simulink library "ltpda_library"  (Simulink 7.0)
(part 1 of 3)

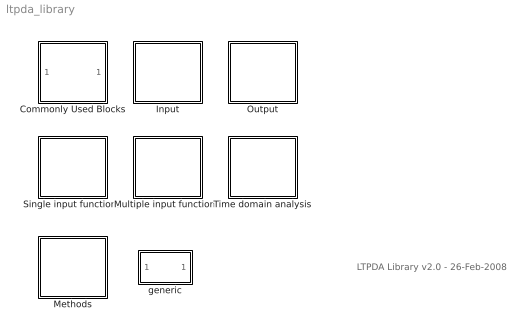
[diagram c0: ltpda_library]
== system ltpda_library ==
  note: LTPDA Library v2.0 - 26-Feb-2008
  Commonly Used Blocks : Subsystem
  Input : Subsystem
  Methods : Subsystem  Tag=subsystem  AncestorBlock=libraryBase/SubSystName
  Multiple input functions : Subsystem
  Output : Subsystem
  Single input functions : Subsystem
  Time domain analysis : Subsystem
  generic : Subsystem  Tag=function

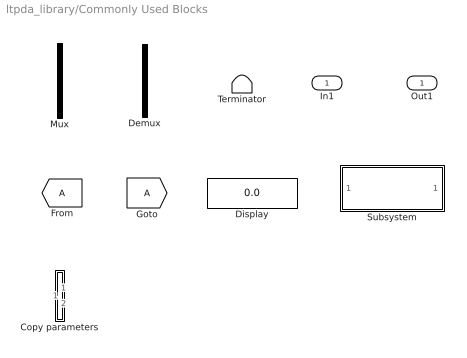
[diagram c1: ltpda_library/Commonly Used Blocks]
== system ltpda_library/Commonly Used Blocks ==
  In1 : Inport  OutDataType=sfix(16)  OutScaling=2^0
  Copy parameters : Subsystem
  Demux : Demux  Tag=demux  Outputs=2
  Display : Display
  Mux : Mux  Tag=mux  Inputs=2
  Subsystem : Subsystem
  Terminator : Terminator
  Out1 : Outport  OutDataType=sfix(16)  OutScaling=2^0

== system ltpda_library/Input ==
  AO from plist : Subsystem  Tag=freepl
  Object from list : Subsystem  Tag=input

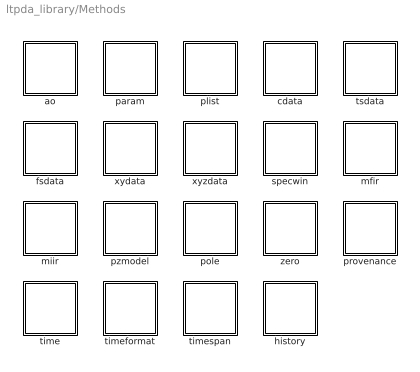
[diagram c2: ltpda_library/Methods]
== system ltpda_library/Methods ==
  ao : Subsystem  Tag=subsystem  AncestorBlock=libraryBase/SubSystName
  cdata : Subsystem  Tag=subsystem  AncestorBlock=libraryBase/SubSystName
  fsdata : Subsystem  Tag=subsystem  AncestorBlock=libraryBase/SubSystName
  history : Subsystem  Tag=subsystem  AncestorBlock=libraryBase/SubSystName
  mfir : Subsystem  Tag=subsystem  AncestorBlock=libraryBase/SubSystName
  miir : Subsystem  Tag=subsystem  AncestorBlock=libraryBase/SubSystName
  param : Subsystem  Tag=subsystem  AncestorBlock=libraryBase/SubSystName
  plist : Subsystem  Tag=subsystem  AncestorBlock=libraryBase/SubSystName
  pole : Subsystem  Tag=subsystem  AncestorBlock=libraryBase/SubSystName
  provenance : Subsystem  Tag=subsystem  AncestorBlock=libraryBase/SubSystName
  pzmodel : Subsystem  Tag=subsystem  AncestorBlock=libraryBase/SubSystName
  specwin : Subsystem  Tag=subsystem  AncestorBlock=libraryBase/SubSystName
  time : Subsystem  Tag=subsystem  AncestorBlock=libraryBase/SubSystName
  timeformat : Subsystem  Tag=subsystem  AncestorBlock=libraryBase/SubSystName
  timespan : Subsystem  Tag=subsystem  AncestorBlock=libraryBase/SubSystName
  tsdata : Subsystem  Tag=subsystem  AncestorBlock=libraryBase/SubSystName
  xydata : Subsystem  Tag=subsystem  AncestorBlock=libraryBase/SubSystName
  xyzdata : Subsystem  Tag=subsystem  AncestorBlock=libraryBase/SubSystName
  zero : Subsystem  Tag=subsystem  AncestorBlock=libraryBase/SubSystName

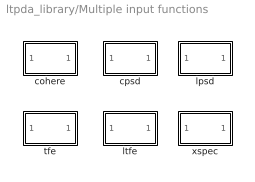
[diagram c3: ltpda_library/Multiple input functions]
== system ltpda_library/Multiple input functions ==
  cohere : Subsystem  Tag=function
  cpsd : Subsystem  Tag=function
  lpsd : Subsystem  Tag=function
  ltfe : Subsystem  Tag=function
  tfe : Subsystem  Tag=function
  xspec : Subsystem  Tag=function

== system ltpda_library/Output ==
  Plot : Subsystem
  Save Result : Subsystem
  iPlot : Subsystem

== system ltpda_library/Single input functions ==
  compute_f : Subsystem  Tag=function
  linedetect : Subsystem  Tag=function
  nfest : Subsystem  Tag=function
  psd : Subsystem  Tag=function
  pwelch : Subsystem  Tag=function
  rms : Subsystem  Tag=function

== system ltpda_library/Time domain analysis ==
  chkts : Subsystem  Tag=function
  polydetrend : Subsystem  Tag=function
  timedomainfit : Subsystem  Tag=function

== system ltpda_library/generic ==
  In1 : Inport  OutDataType=sfix(16)  OutScaling=2^0
  generic : M-S-Function  Tag=generic  FunctionName=ltpdasim
  Out1 : Outport  OutDataType=sfix(16)  OutScaling=2^0
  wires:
  generic/1 -> Out1/1
  In1/1 -> generic/1

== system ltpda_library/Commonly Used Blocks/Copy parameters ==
  In1 : Inport  OutDataType=sfix(16)  OutScaling=2^0
  In2 : Inport  Port=2  OutDataType=sfix(16)  OutScaling=2^0
  copyparam : M-S-Function  FunctionName=g_copyparams
  Out1 : Outport  OutDataType=sfix(16)  OutScaling=2^0
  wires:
  copyparam/1 -> Out1/1
  In1/1 -> copyparam/1
  In2/1 -> copyparam/2

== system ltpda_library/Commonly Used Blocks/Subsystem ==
  In1 : Inport  OutDataType=sfix(16)  OutScaling=2^0
  Out1 : Outport  OutDataType=sfix(16)  OutScaling=2^0
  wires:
  In1/1 -> Out1/1

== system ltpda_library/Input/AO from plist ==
  pl2ao : M-S-Function  FunctionName=g_pl2ao
  Out1 : Outport  OutDataType=sfix(16)  OutScaling=2^0
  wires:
  pl2ao/1 -> Out1/1

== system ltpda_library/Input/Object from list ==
  Input : Constant  Value=0  OutDataType=sfix(16)  OutScaling=2^0
  Input AO : Outport  OutDataType=sfix(16)  OutScaling=2^0
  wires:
  Input/1 -> Input AO/1

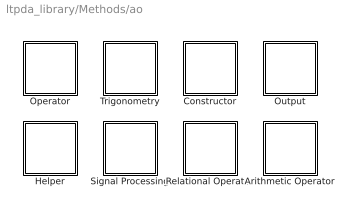
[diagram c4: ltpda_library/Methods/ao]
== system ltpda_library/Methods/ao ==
  Arithmetic Operator : Subsystem  Tag=subsystem  AncestorBlock=libraryBase/SubSystName
  Constructor : Subsystem  Tag=subsystem  AncestorBlock=libraryBase/SubSystName
  Helper : Subsystem  Tag=subsystem  AncestorBlock=libraryBase/SubSystName
  Operator : Subsystem  Tag=subsystem  AncestorBlock=libraryBase/SubSystName
  Output : Subsystem  Tag=subsystem  AncestorBlock=libraryBase/SubSystName
  Relational Operator : Subsystem  Tag=subsystem  AncestorBlock=libraryBase/SubSystName
  Signal Processing : Subsystem  Tag=subsystem  AncestorBlock=libraryBase/SubSystName
  Trigonometry : Subsystem  Tag=subsystem  AncestorBlock=libraryBase/SubSystName

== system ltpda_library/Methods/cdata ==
  Constructor : Subsystem  Tag=subsystem  AncestorBlock=libraryBase/SubSystName
  Helper : Subsystem  Tag=subsystem  AncestorBlock=libraryBase/SubSystName
  Output : Subsystem  Tag=subsystem  AncestorBlock=libraryBase/SubSystName
  Relational Operator : Subsystem  Tag=subsystem  AncestorBlock=libraryBase/SubSystName

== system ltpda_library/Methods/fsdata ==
  Constructor : Subsystem  Tag=subsystem  AncestorBlock=libraryBase/SubSystName
  Helper : Subsystem  Tag=subsystem  AncestorBlock=libraryBase/SubSystName
  Output : Subsystem  Tag=subsystem  AncestorBlock=libraryBase/SubSystName
  Relational Operator : Subsystem  Tag=subsystem  AncestorBlock=libraryBase/SubSystName

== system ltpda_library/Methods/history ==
  Constructor : Subsystem  Tag=subsystem  AncestorBlock=libraryBase/SubSystName
  Helper : Subsystem  Tag=subsystem  AncestorBlock=libraryBase/SubSystName
  Output : Subsystem  Tag=subsystem  AncestorBlock=libraryBase/SubSystName
  Relational Operator : Subsystem  Tag=subsystem  AncestorBlock=libraryBase/SubSystName

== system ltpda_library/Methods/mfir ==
  Constructor : Subsystem  Tag=subsystem  AncestorBlock=libraryBase/SubSystName
  Helper : Subsystem  Tag=subsystem  AncestorBlock=libraryBase/SubSystName
  Output : Subsystem  Tag=subsystem  AncestorBlock=libraryBase/SubSystName
  Relational Operator : Subsystem  Tag=subsystem  AncestorBlock=libraryBase/SubSystName
  Signal Processing : Subsystem  Tag=subsystem  AncestorBlock=libraryBase/SubSystName

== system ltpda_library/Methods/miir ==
  Constructor : Subsystem  Tag=subsystem  AncestorBlock=libraryBase/SubSystName
  Helper : Subsystem  Tag=subsystem  AncestorBlock=libraryBase/SubSystName
  Output : Subsystem  Tag=subsystem  AncestorBlock=libraryBase/SubSystName
  Relational Operator : Subsystem  Tag=subsystem  AncestorBlock=libraryBase/SubSystName
  Signal Processing : Subsystem  Tag=subsystem  AncestorBlock=libraryBase/SubSystName

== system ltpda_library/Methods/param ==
  Constructor : Subsystem  Tag=subsystem  AncestorBlock=libraryBase/SubSystName
  Helper : Subsystem  Tag=subsystem  AncestorBlock=libraryBase/SubSystName
  Operator : Subsystem  Tag=subsystem  AncestorBlock=libraryBase/SubSystName
  Output : Subsystem  Tag=subsystem  AncestorBlock=libraryBase/SubSystName
  Relational Operator : Subsystem  Tag=subsystem  AncestorBlock=libraryBase/SubSystName

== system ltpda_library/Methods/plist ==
  Constructor : Subsystem  Tag=subsystem  AncestorBlock=libraryBase/SubSystName
  Helper : Subsystem  Tag=subsystem  AncestorBlock=libraryBase/SubSystName
  Output : Subsystem  Tag=subsystem  AncestorBlock=libraryBase/SubSystName
  Relational Operator : Subsystem  Tag=subsystem  AncestorBlock=libraryBase/SubSystName
  Signal Processing : Subsystem  Tag=subsystem  AncestorBlock=libraryBase/SubSystName

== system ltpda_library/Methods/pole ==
  Constructor : Subsystem  Tag=subsystem  AncestorBlock=libraryBase/SubSystName
  Helper : Subsystem  Tag=subsystem  AncestorBlock=libraryBase/SubSystName
  Output : Subsystem  Tag=subsystem  AncestorBlock=libraryBase/SubSystName
  Relational Operator : Subsystem  Tag=subsystem  AncestorBlock=libraryBase/SubSystName
  Signal Processing : Subsystem  Tag=subsystem  AncestorBlock=libraryBase/SubSystName

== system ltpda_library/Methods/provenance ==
  Constructor : Subsystem  Tag=subsystem  AncestorBlock=libraryBase/SubSystName
  Helper : Subsystem  Tag=subsystem  AncestorBlock=libraryBase/SubSystName
  Output : Subsystem  Tag=subsystem  AncestorBlock=libraryBase/SubSystName
  Relational Operator : Subsystem  Tag=subsystem  AncestorBlock=libraryBase/SubSystName

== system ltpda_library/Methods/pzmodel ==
  Constructor : Subsystem  Tag=subsystem  AncestorBlock=libraryBase/SubSystName
  Helper : Subsystem  Tag=subsystem  AncestorBlock=libraryBase/SubSystName
  Operator : Subsystem  Tag=subsystem  AncestorBlock=libraryBase/SubSystName
  Output : Subsystem  Tag=subsystem  AncestorBlock=libraryBase/SubSystName
  Relational Operator : Subsystem  Tag=subsystem  AncestorBlock=libraryBase/SubSystName
  Signal Processing : Subsystem  Tag=subsystem  AncestorBlock=libraryBase/SubSystName

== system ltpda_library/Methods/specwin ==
  Constructor : Subsystem  Tag=subsystem  AncestorBlock=libraryBase/SubSystName
  Helper : Subsystem  Tag=subsystem  AncestorBlock=libraryBase/SubSystName
  Output : Subsystem  Tag=subsystem  AncestorBlock=libraryBase/SubSystName
  Relational Operator : Subsystem  Tag=subsystem  AncestorBlock=libraryBase/SubSystName

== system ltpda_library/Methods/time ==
  Arithmetic Operator : Subsystem  Tag=subsystem  AncestorBlock=libraryBase/SubSystName
  Constructor : Subsystem  Tag=subsystem  AncestorBlock=libraryBase/SubSystName
  Helper : Subsystem  Tag=subsystem  AncestorBlock=libraryBase/SubSystName
  Output : Subsystem  Tag=subsystem  AncestorBlock=libraryBase/SubSystName
  Relational Operator : Subsystem  Tag=subsystem  AncestorBlock=libraryBase/SubSystName

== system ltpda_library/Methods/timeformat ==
  Constructor : Subsystem  Tag=subsystem  AncestorBlock=libraryBase/SubSystName
  Helper : Subsystem  Tag=subsystem  AncestorBlock=libraryBase/SubSystName
  Output : Subsystem  Tag=subsystem  AncestorBlock=libraryBase/SubSystName
  Relational Operator : Subsystem  Tag=subsystem  AncestorBlock=libraryBase/SubSystName

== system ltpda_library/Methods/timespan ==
  Constructor : Subsystem  Tag=subsystem  AncestorBlock=libraryBase/SubSystName
  Helper : Subsystem  Tag=subsystem  AncestorBlock=libraryBase/SubSystName
  Output : Subsystem  Tag=subsystem  AncestorBlock=libraryBase/SubSystName
  Relational Operator : Subsystem  Tag=subsystem  AncestorBlock=libraryBase/SubSystName

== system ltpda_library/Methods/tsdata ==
  Constructor : Subsystem  Tag=subsystem  AncestorBlock=libraryBase/SubSystName
  Helper : Subsystem  Tag=subsystem  AncestorBlock=libraryBase/SubSystName
  Output : Subsystem  Tag=subsystem  AncestorBlock=libraryBase/SubSystName
  Relational Operator : Subsystem  Tag=subsystem  AncestorBlock=libraryBase/SubSystName

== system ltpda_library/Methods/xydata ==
  Constructor : Subsystem  Tag=subsystem  AncestorBlock=libraryBase/SubSystName
  Helper : Subsystem  Tag=subsystem  AncestorBlock=libraryBase/SubSystName
  Output : Subsystem  Tag=subsystem  AncestorBlock=libraryBase/SubSystName
  Relational Operator : Subsystem  Tag=subsystem  AncestorBlock=libraryBase/SubSystName

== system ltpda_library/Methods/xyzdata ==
  Constructor : Subsystem  Tag=subsystem  AncestorBlock=libraryBase/SubSystName
  Helper : Subsystem  Tag=subsystem  AncestorBlock=libraryBase/SubSystName
  Output : Subsystem  Tag=subsystem  AncestorBlock=libraryBase/SubSystName
  Relational Operator : Subsystem  Tag=subsystem  AncestorBlock=libraryBase/SubSystName

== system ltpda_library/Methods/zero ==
  Constructor : Subsystem  Tag=subsystem  AncestorBlock=libraryBase/SubSystName
  Helper : Subsystem  Tag=subsystem  AncestorBlock=libraryBase/SubSystName
  Output : Subsystem  Tag=subsystem  AncestorBlock=libraryBase/SubSystName
  Relational Operator : Subsystem  Tag=subsystem  AncestorBlock=libraryBase/SubSystName
  Signal Processing : Subsystem  Tag=subsystem  AncestorBlock=libraryBase/SubSystName

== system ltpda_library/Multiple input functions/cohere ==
  In1 : Inport  OutDataType=sfix(16)  OutScaling=2^0
  ltpda_cohere : M-S-Function  Tag=ltpda_cohere  FunctionName=ltpdasim
  Out1 : Outport  OutDataType=sfix(16)  OutScaling=2^0
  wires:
  ltpda_cohere/1 -> Out1/1
  In1/1 -> ltpda_cohere/1

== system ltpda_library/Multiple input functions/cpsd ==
  In1 : Inport  OutDataType=sfix(16)  OutScaling=2^0
  ltpda_cpsd : M-S-Function  Tag=ltpda_cpsd  FunctionName=ltpdasim
  Out1 : Outport  OutDataType=sfix(16)  OutScaling=2^0
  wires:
  ltpda_cpsd/1 -> Out1/1
  In1/1 -> ltpda_cpsd/1

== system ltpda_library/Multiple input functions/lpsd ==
  In1 : Inport  OutDataType=sfix(16)  OutScaling=2^0
  ltpda_lpsd : M-S-Function  Tag=ltpda_lpsd  FunctionName=ltpdasim
  Out1 : Outport  OutDataType=sfix(16)  OutScaling=2^0
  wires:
  In1/1 -> ltpda_lpsd/1
  ltpda_lpsd/1 -> Out1/1

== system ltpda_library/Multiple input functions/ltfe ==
  In1 : Inport  OutDataType=sfix(16)  OutScaling=2^0
  ltpda_ltfe : M-S-Function  Tag=ltpda_ltfe  FunctionName=ltpdasim
  Out1 : Outport  OutDataType=sfix(16)  OutScaling=2^0
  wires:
  In1/1 -> ltpda_ltfe/1
  ltpda_ltfe/1 -> Out1/1

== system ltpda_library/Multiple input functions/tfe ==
  In1 : Inport  OutDataType=sfix(16)  OutScaling=2^0
  ltpda_tfe : M-S-Function  Tag=ltpda_tfe  FunctionName=ltpdasim
  Out1 : Outport  OutDataType=sfix(16)  OutScaling=2^0
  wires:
  ltpda_tfe/1 -> Out1/1
  In1/1 -> ltpda_tfe/1

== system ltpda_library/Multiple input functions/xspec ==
  In1 : Inport  OutDataType=sfix(16)  OutScaling=2^0
  ltpda_xspec : M-S-Function  Tag=ltpda_xspec  FunctionName=ltpdasim
  Out1 : Outport  OutDataType=sfix(16)  OutScaling=2^0
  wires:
  ltpda_xspec/1 -> Out1/1
  In1/1 -> ltpda_xspec/1

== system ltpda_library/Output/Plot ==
  In1 : Inport  OutDataType=sfix(16)  OutScaling=2^0
  plot : M-S-Function  FunctionName=g_plot
  Out1 : Outport  OutDataType=sfix(16)  OutScaling=2^0
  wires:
  plot/1 -> Out1/1
  In1/1 -> plot/1

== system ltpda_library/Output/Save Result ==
  In1 : Inport  OutDataType=sfix(16)  OutScaling=2^0
  save result : M-S-Function  FunctionName=g_saveresult
  Out1 : Outport  OutDataType=sfix(16)  OutScaling=2^0
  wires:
  In1/1 -> save result/1
  save result/1 -> Out1/1

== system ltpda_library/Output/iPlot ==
  In1 : Inport  OutDataType=sfix(16)  OutScaling=2^0
  iplot : M-S-Function  FunctionName=g_iplot
  Out1 : Outport  OutDataType=sfix(16)  OutScaling=2^0
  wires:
  In1/1 -> iplot/1
  iplot/1 -> Out1/1

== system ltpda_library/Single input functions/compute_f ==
  In1 : Inport  OutDataType=sfix(16)  OutScaling=2^0
  ltpda_compute_f : M-S-Function  Tag=ltpda_compute_f  FunctionName=ltpdasim
  Out1 : Outport  OutDataType=sfix(16)  OutScaling=2^0
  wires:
  ltpda_compute_f/1 -> Out1/1
  In1/1 -> ltpda_compute_f/1

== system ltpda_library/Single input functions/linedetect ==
  In1 : Inport  OutDataType=sfix(16)  OutScaling=2^0
  ltpda_linedetect : M-S-Function  Tag=ltpda_linedetect  FunctionName=ltpdasim
  Out1 : Outport  OutDataType=sfix(16)  OutScaling=2^0
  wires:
  In1/1 -> ltpda_linedetect/1
  ltpda_linedetect/1 -> Out1/1

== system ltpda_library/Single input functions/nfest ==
  In1 : Inport  OutDataType=sfix(16)  OutScaling=2^0
  ltpda_nfest : M-S-Function  Tag=ltpda_nfest  FunctionName=ltpdasim
  Out1 : Outport  OutDataType=sfix(16)  OutScaling=2^0
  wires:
  ltpda_nfest/1 -> Out1/1
  In1/1 -> ltpda_nfest/1

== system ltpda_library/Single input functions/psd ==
  In1 : Inport  OutDataType=sfix(16)  OutScaling=2^0
  ltpda_psd : M-S-Function  Tag=ltpda_psd  FunctionName=ltpdasim
  Out1 : Outport  OutDataType=sfix(16)  OutScaling=2^0
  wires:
  ltpda_psd/1 -> Out1/1
  In1/1 -> ltpda_psd/1

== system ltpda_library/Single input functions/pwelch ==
  In1 : Inport  OutDataType=sfix(16)  OutScaling=2^0
  ltpda_pwelch : M-S-Function  Tag=ltpda_pwelch  FunctionName=ltpdasim
  Out1 : Outport  OutDataType=sfix(16)  OutScaling=2^0
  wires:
  In1/1 -> ltpda_pwelch/1
  ltpda_pwelch/1 -> Out1/1

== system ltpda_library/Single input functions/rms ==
  In1 : Inport  OutDataType=sfix(16)  OutScaling=2^0
  ltpda_rms : M-S-Function  Tag=ltpda_rms  FunctionName=ltpdasim
  Out1 : Outport  OutDataType=sfix(16)  OutScaling=2^0
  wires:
  In1/1 -> ltpda_rms/1
  ltpda_rms/1 -> Out1/1

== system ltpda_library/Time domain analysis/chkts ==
  In1 : Inport  OutDataType=sfix(16)  OutScaling=2^0
  ltpda_chkts : M-S-Function  Tag=ltpda_chkts  FunctionName=ltpdasim
  Out1 : Outport  OutDataType=sfix(16)  OutScaling=2^0
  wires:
  ltpda_chkts/1 -> Out1/1
  In1/1 -> ltpda_chkts/1

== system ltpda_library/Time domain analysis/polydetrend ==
  In1 : Inport  OutDataType=sfix(16)  OutScaling=2^0
  ltpda_polydetrend : M-S-Function  Tag=ltpda_polydetrend  FunctionName=ltpdasim
  Out1 : Outport  OutDataType=sfix(16)  OutScaling=2^0
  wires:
  In1/1 -> ltpda_polydetrend/1
  ltpda_polydetrend/1 -> Out1/1

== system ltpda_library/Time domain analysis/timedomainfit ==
  In1 : Inport  OutDataType=sfix(16)  OutScaling=2^0
  ltpda_timedomainfit : M-S-Function  Tag=ltpda_timedomainfit  FunctionName=ltpdasim
  Out1 : Outport  OutDataType=sfix(16)  OutScaling=2^0
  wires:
  ltpda_timedomainfit/1 -> Out1/1
  In1/1 -> ltpda_timedomainfit/1

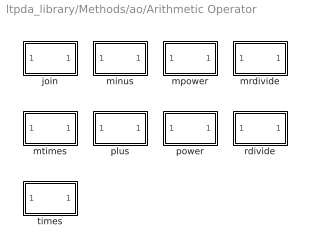
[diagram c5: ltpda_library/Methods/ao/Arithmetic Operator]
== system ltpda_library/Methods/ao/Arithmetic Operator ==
  join : Subsystem  Tag=method ao  AncestorBlock=libraryBase/function
  minus : Subsystem  Tag=method ao  AncestorBlock=libraryBase/function
  mpower : Subsystem  Tag=method ao  AncestorBlock=libraryBase/function
  mrdivide : Subsystem  Tag=method ao  AncestorBlock=libraryBase/function
  mtimes : Subsystem  Tag=method ao  AncestorBlock=libraryBase/function
  plus : Subsystem  Tag=method ao  AncestorBlock=libraryBase/function
  power : Subsystem  Tag=method ao  AncestorBlock=libraryBase/function
  rdivide : Subsystem  Tag=method ao  AncestorBlock=libraryBase/function
  times : Subsystem  Tag=method ao  AncestorBlock=libraryBase/function

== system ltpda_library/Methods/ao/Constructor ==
  ao : Subsystem  Tag=method ao  AncestorBlock=libraryBase/constructor

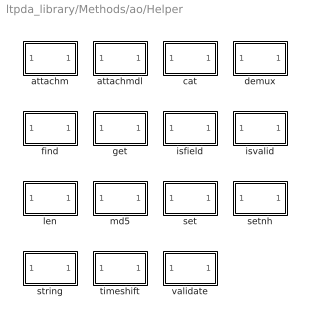
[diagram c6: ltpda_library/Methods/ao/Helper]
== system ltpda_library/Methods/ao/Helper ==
  attachm : Subsystem  Tag=method ao  AncestorBlock=libraryBase/function
  attachmdl : Subsystem  Tag=method ao  AncestorBlock=libraryBase/function
  cat : Subsystem  Tag=method ao  AncestorBlock=libraryBase/function
  demux : Subsystem  Tag=method ao  AncestorBlock=libraryBase/function
  find : Subsystem  Tag=method ao  AncestorBlock=libraryBase/function
  get : Subsystem  Tag=method ao  AncestorBlock=libraryBase/function
  isfield : Subsystem  Tag=method ao  AncestorBlock=libraryBase/function
  isvalid : Subsystem  Tag=method ao  AncestorBlock=libraryBase/function
  len : Subsystem  Tag=method ao  AncestorBlock=libraryBase/function
  md5 : Subsystem  Tag=method ao  AncestorBlock=libraryBase/function
  set : Subsystem  Tag=method ao  AncestorBlock=libraryBase/function
  setnh : Subsystem  Tag=method ao  AncestorBlock=libraryBase/function
  string : Subsystem  Tag=method ao  AncestorBlock=libraryBase/function
  timeshift : Subsystem  Tag=method ao  AncestorBlock=libraryBase/function
  validate : Subsystem  Tag=method ao  AncestorBlock=libraryBase/function

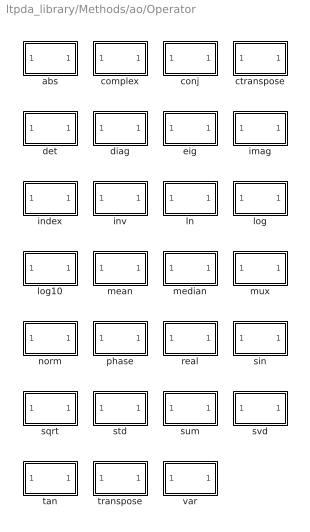
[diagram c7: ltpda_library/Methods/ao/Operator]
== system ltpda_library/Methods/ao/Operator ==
  abs : Subsystem  Tag=method ao  AncestorBlock=libraryBase/function
  complex : Subsystem  Tag=method ao  AncestorBlock=libraryBase/function
  conj : Subsystem  Tag=method ao  AncestorBlock=libraryBase/function
  ctranspose : Subsystem  Tag=method ao  AncestorBlock=libraryBase/function
  det : Subsystem  Tag=method ao  AncestorBlock=libraryBase/function
  diag : Subsystem  Tag=method ao  AncestorBlock=libraryBase/function
  eig : Subsystem  Tag=method ao  AncestorBlock=libraryBase/function
  imag : Subsystem  Tag=method ao  AncestorBlock=libraryBase/function
  index : Subsystem  Tag=method ao  AncestorBlock=libraryBase/function
  inv : Subsystem  Tag=method ao  AncestorBlock=libraryBase/function
  ln : Subsystem  Tag=method ao  AncestorBlock=libraryBase/function
  log : Subsystem  Tag=method ao  AncestorBlock=libraryBase/function
  log10 : Subsystem  Tag=method ao  AncestorBlock=libraryBase/function
  mean : Subsystem  Tag=method ao  AncestorBlock=libraryBase/function
  median : Subsystem  Tag=method ao  AncestorBlock=libraryBase/function
  mux : Subsystem  Tag=method ao  AncestorBlock=libraryBase/function
  norm : Subsystem  Tag=method ao  AncestorBlock=libraryBase/function
  phase : Subsystem  Tag=method ao  AncestorBlock=libraryBase/function
  real : Subsystem  Tag=method ao  AncestorBlock=libraryBase/function
  sin : Subsystem  Tag=method ao  AncestorBlock=libraryBase/function
  sqrt : Subsystem  Tag=method ao  AncestorBlock=libraryBase/function
  std : Subsystem  Tag=method ao  AncestorBlock=libraryBase/function
  sum : Subsystem  Tag=method ao  AncestorBlock=libraryBase/function
  svd : Subsystem  Tag=method ao  AncestorBlock=libraryBase/function
  tan : Subsystem  Tag=method ao  AncestorBlock=libraryBase/function
  transpose : Subsystem  Tag=method ao  AncestorBlock=libraryBase/function
  var : Subsystem  Tag=method ao  AncestorBlock=libraryBase/function

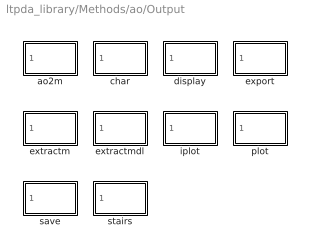
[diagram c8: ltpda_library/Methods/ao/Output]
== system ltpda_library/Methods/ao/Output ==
  ao2m : Subsystem  Tag=method ao  AncestorBlock=libraryBase/output
  char : Subsystem  Tag=method ao  AncestorBlock=libraryBase/output
  display : Subsystem  Tag=method ao  AncestorBlock=libraryBase/output
  export : Subsystem  Tag=method ao  AncestorBlock=libraryBase/output
  extractm : Subsystem  Tag=method ao  AncestorBlock=libraryBase/output
  extractmdl : Subsystem  Tag=method ao  AncestorBlock=libraryBase/output
  iplot : Subsystem  Tag=method ao  AncestorBlock=libraryBase/output
  plot : Subsystem  Tag=method ao  AncestorBlock=libraryBase/output
  save : Subsystem  Tag=method ao  AncestorBlock=libraryBase/output
  stairs : Subsystem  Tag=method ao  AncestorBlock=libraryBase/output

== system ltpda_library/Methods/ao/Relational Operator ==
  eq : Subsystem  Tag=method ao  AncestorBlock=libraryBase/function
  ge : Subsystem  Tag=method ao  AncestorBlock=libraryBase/function
  gt : Subsystem  Tag=method ao  AncestorBlock=libraryBase/function
  le : Subsystem  Tag=method ao  AncestorBlock=libraryBase/function
  lt : Subsystem  Tag=method ao  AncestorBlock=libraryBase/function
  ne : Subsystem  Tag=method ao  AncestorBlock=libraryBase/function

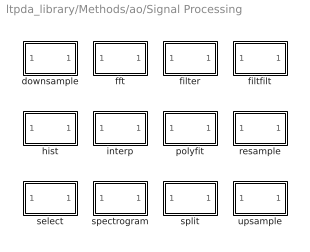
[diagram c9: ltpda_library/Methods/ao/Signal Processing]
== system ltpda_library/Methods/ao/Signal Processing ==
  downsample : Subsystem  Tag=method ao  AncestorBlock=libraryBase/function
  fft : Subsystem  Tag=method ao  AncestorBlock=libraryBase/function
  filter : Subsystem  Tag=method ao  AncestorBlock=libraryBase/function
  filtfilt : Subsystem  Tag=method ao  AncestorBlock=libraryBase/function
  hist : Subsystem  Tag=method ao  AncestorBlock=libraryBase/function
  interp : Subsystem  Tag=method ao  AncestorBlock=libraryBase/function
  polyfit : Subsystem  Tag=method ao  AncestorBlock=libraryBase/function
  resample : Subsystem  Tag=method ao  AncestorBlock=libraryBase/function
  select : Subsystem  Tag=method ao  AncestorBlock=libraryBase/function
  spectrogram : Subsystem  Tag=method ao  AncestorBlock=libraryBase/function
  split : Subsystem  Tag=method ao  AncestorBlock=libraryBase/function
  upsample : Subsystem  Tag=method ao  AncestorBlock=libraryBase/function

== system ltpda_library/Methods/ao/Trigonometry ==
  acos : Subsystem  Tag=method ao  AncestorBlock=libraryBase/function
  asin : Subsystem  Tag=method ao  AncestorBlock=libraryBase/function
  atan : Subsystem  Tag=method ao  AncestorBlock=libraryBase/function
  cos : Subsystem  Tag=method ao  AncestorBlock=libraryBase/function
  exp : Subsystem  Tag=method ao  AncestorBlock=libraryBase/function

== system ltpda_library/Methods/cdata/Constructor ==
  cdata : Subsystem  Tag=method cdata  AncestorBlock=libraryBase/constructor

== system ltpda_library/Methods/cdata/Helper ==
  get : Subsystem  Tag=method cdata  AncestorBlock=libraryBase/function
  isfield : Subsystem  Tag=method cdata  AncestorBlock=libraryBase/function
  isvalid : Subsystem  Tag=method cdata  AncestorBlock=libraryBase/function
  set : Subsystem  Tag=method cdata  AncestorBlock=libraryBase/function

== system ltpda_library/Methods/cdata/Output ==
  char : Subsystem  Tag=method cdata  AncestorBlock=libraryBase/output
  display : Subsystem  Tag=method cdata  AncestorBlock=libraryBase/output
  save : Subsystem  Tag=method cdata  AncestorBlock=libraryBase/output

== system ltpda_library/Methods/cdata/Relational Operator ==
  eq : Subsystem  Tag=method cdata  AncestorBlock=libraryBase/function
  ne : Subsystem  Tag=method cdata  AncestorBlock=libraryBase/function

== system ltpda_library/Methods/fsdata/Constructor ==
  fsdata : Subsystem  Tag=method fsdata  AncestorBlock=libraryBase/constructor

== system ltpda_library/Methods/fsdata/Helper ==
  get : Subsystem  Tag=method fsdata  AncestorBlock=libraryBase/function
  isfield : Subsystem  Tag=method fsdata  AncestorBlock=libraryBase/function
  isvalid : Subsystem  Tag=method fsdata  AncestorBlock=libraryBase/function
  set : Subsystem  Tag=method fsdata  AncestorBlock=libraryBase/function

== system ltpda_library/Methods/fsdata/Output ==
  char : Subsystem  Tag=method fsdata  AncestorBlock=libraryBase/output
  display : Subsystem  Tag=method fsdata  AncestorBlock=libraryBase/output
  save : Subsystem  Tag=method fsdata  AncestorBlock=libraryBase/output

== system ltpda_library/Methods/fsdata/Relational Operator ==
  eq : Subsystem  Tag=method fsdata  AncestorBlock=libraryBase/function
  ne : Subsystem  Tag=method fsdata  AncestorBlock=libraryBase/function

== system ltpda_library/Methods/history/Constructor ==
  history : Subsystem  Tag=method history  AncestorBlock=libraryBase/constructor

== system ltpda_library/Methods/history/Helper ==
  get : Subsystem  Tag=method history  AncestorBlock=libraryBase/function
  isfield : Subsystem  Tag=method history  AncestorBlock=libraryBase/function
  isvalid : Subsystem  Tag=method history  AncestorBlock=libraryBase/function
  set : Subsystem  Tag=method history  AncestorBlock=libraryBase/function

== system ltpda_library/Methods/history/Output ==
  char : Subsystem  Tag=method history  AncestorBlock=libraryBase/output
  display : Subsystem  Tag=method history  AncestorBlock=libraryBase/output
  hist2dot : Subsystem  Tag=method history  AncestorBlock=libraryBase/output
  plot : Subsystem  Tag=method history  AncestorBlock=libraryBase/output
  save : Subsystem  Tag=method history  AncestorBlock=libraryBase/output
  string : Subsystem  Tag=method history  AncestorBlock=libraryBase/output

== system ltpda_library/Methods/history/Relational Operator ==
  eq : Subsystem  Tag=method history  AncestorBlock=libraryBase/function
  ne : Subsystem  Tag=method history  AncestorBlock=libraryBase/function

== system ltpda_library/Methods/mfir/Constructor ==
  mfir : Subsystem  Tag=method mfir  AncestorBlock=libraryBase/constructor

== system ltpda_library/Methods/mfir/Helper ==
  get : Subsystem  Tag=method mfir  AncestorBlock=libraryBase/function
  isfield : Subsystem  Tag=method mfir  AncestorBlock=libraryBase/function
  isvalid : Subsystem  Tag=method mfir  AncestorBlock=libraryBase/function
  redesign : Subsystem  Tag=method mfir  AncestorBlock=libraryBase/function
  set : Subsystem  Tag=method mfir  AncestorBlock=libraryBase/function
  string : Subsystem  Tag=method mfir  AncestorBlock=libraryBase/function

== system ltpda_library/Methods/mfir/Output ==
  char : Subsystem  Tag=method mfir  AncestorBlock=libraryBase/output
  display : Subsystem  Tag=method mfir  AncestorBlock=libraryBase/output
  save : Subsystem  Tag=method mfir  AncestorBlock=libraryBase/output

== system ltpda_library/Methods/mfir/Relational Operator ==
  eq : Subsystem  Tag=method mfir  AncestorBlock=libraryBase/function
  ne : Subsystem  Tag=method mfir  AncestorBlock=libraryBase/function

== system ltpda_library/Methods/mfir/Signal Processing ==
  resp : Subsystem  Tag=method mfir  AncestorBlock=libraryBase/function

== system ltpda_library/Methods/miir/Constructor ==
  miir : Subsystem  Tag=method miir  AncestorBlock=libraryBase/constructor

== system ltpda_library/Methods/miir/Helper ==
  get : Subsystem  Tag=method miir  AncestorBlock=libraryBase/function
  isfield : Subsystem  Tag=method miir  AncestorBlock=libraryBase/function
  isvalid : Subsystem  Tag=method miir  AncestorBlock=libraryBase/function
  redesign : Subsystem  Tag=method miir  AncestorBlock=libraryBase/function
  set : Subsystem  Tag=method miir  AncestorBlock=libraryBase/function

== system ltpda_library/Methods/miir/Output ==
  char : Subsystem  Tag=method miir  AncestorBlock=libraryBase/output
  display : Subsystem  Tag=method miir  AncestorBlock=libraryBase/output
  save : Subsystem  Tag=method miir  AncestorBlock=libraryBase/output
  string : Subsystem  Tag=method miir  AncestorBlock=libraryBase/output

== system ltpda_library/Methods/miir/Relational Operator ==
  eq : Subsystem  Tag=method miir  AncestorBlock=libraryBase/function
  ne : Subsystem  Tag=method miir  AncestorBlock=libraryBase/function

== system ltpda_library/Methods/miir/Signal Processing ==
  resp : Subsystem  Tag=method miir  AncestorBlock=libraryBase/function

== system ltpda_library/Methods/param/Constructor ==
  param : Subsystem  Tag=method param  AncestorBlock=libraryBase/constructor

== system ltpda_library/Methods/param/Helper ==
  cat : Subsystem  Tag=method param  AncestorBlock=libraryBase/function
  get : Subsystem  Tag=method param  AncestorBlock=libraryBase/function
  isfield : Subsystem  Tag=method param  AncestorBlock=libraryBase/function
  isvalid : Subsystem  Tag=method param  AncestorBlock=libraryBase/function
  set : Subsystem  Tag=method param  AncestorBlock=libraryBase/function

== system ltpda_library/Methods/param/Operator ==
  mux : Subsystem  Tag=method param  AncestorBlock=libraryBase/function

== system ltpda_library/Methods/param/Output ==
  char : Subsystem  Tag=method param  AncestorBlock=libraryBase/output
  display : Subsystem  Tag=method param  AncestorBlock=libraryBase/output
  save : Subsystem  Tag=method param  AncestorBlock=libraryBase/output
  string : Subsystem  Tag=method param  AncestorBlock=libraryBase/output

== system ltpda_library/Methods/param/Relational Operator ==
  eq : Subsystem  Tag=method param  AncestorBlock=libraryBase/function
  ne : Subsystem  Tag=method param  AncestorBlock=libraryBase/function

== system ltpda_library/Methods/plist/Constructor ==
  plist : Subsystem  Tag=method plist  AncestorBlock=libraryBase/constructor

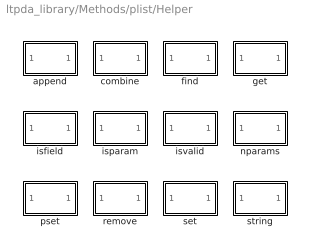
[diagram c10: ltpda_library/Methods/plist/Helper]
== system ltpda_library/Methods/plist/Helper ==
  append : Subsystem  Tag=method plist  AncestorBlock=libraryBase/function
  combine : Subsystem  Tag=method plist  AncestorBlock=libraryBase/function
  find : Subsystem  Tag=method plist  AncestorBlock=libraryBase/function
  get : Subsystem  Tag=method plist  AncestorBlock=libraryBase/function
  isfield : Subsystem  Tag=method plist  AncestorBlock=libraryBase/function
  isparam : Subsystem  Tag=method plist  AncestorBlock=libraryBase/function
  isvalid : Subsystem  Tag=method plist  AncestorBlock=libraryBase/function
  nparams : Subsystem  Tag=method plist  AncestorBlock=libraryBase/function
  pset : Subsystem  Tag=method plist  AncestorBlock=libraryBase/function
  remove : Subsystem  Tag=method plist  AncestorBlock=libraryBase/function
  set : Subsystem  Tag=method plist  AncestorBlock=libraryBase/function
  string : Subsystem  Tag=method plist  AncestorBlock=libraryBase/function

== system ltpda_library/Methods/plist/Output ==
  char : Subsystem  Tag=method plist  AncestorBlock=libraryBase/output
  display : Subsystem  Tag=method plist  AncestorBlock=libraryBase/output
  save : Subsystem  Tag=method plist  AncestorBlock=libraryBase/output

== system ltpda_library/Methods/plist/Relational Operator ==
  eq : Subsystem  Tag=method plist  AncestorBlock=libraryBase/function
  ne : Subsystem  Tag=method plist  AncestorBlock=libraryBase/function

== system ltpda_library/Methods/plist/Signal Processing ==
  pzmresp : Subsystem  Tag=method plist  AncestorBlock=libraryBase/function
  resp : Subsystem  Tag=method plist  AncestorBlock=libraryBase/function

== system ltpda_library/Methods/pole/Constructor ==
  pole : Subsystem  Tag=method pole  AncestorBlock=libraryBase/constructor

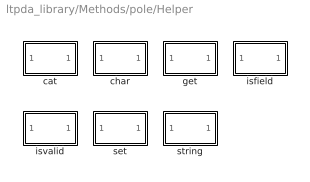
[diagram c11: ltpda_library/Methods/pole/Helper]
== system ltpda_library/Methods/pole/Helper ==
  cat : Subsystem  Tag=method pole  AncestorBlock=libraryBase/function
  char : Subsystem  Tag=method pole  AncestorBlock=libraryBase/function
  get : Subsystem  Tag=method pole  AncestorBlock=libraryBase/function
  isfield : Subsystem  Tag=method pole  AncestorBlock=libraryBase/function
  isvalid : Subsystem  Tag=method pole  AncestorBlock=libraryBase/function
  set : Subsystem  Tag=method pole  AncestorBlock=libraryBase/function
  string : Subsystem  Tag=method pole  AncestorBlock=libraryBase/function

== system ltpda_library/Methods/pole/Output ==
  display : Subsystem  Tag=method pole  AncestorBlock=libraryBase/output
  save : Subsystem  Tag=method pole  AncestorBlock=libraryBase/output

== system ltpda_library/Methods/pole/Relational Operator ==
  eq : Subsystem  Tag=method pole  AncestorBlock=libraryBase/function
  ne : Subsystem  Tag=method pole  AncestorBlock=libraryBase/function

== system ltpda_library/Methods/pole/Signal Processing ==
  resp : Subsystem  Tag=method pole  AncestorBlock=libraryBase/function

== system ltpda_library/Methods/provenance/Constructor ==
  provenance : Subsystem  Tag=method provenance  AncestorBlock=libraryBase/constructor

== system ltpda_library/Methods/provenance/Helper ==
  get : Subsystem  Tag=method provenance  AncestorBlock=libraryBase/function
  isfield : Subsystem  Tag=method provenance  AncestorBlock=libraryBase/function
  isvalid : Subsystem  Tag=method provenance  AncestorBlock=libraryBase/function
  set : Subsystem  Tag=method provenance  AncestorBlock=libraryBase/function

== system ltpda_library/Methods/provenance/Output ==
  char : Subsystem  Tag=method provenance  AncestorBlock=libraryBase/output
  display : Subsystem  Tag=method provenance  AncestorBlock=libraryBase/output
  save : Subsystem  Tag=method provenance  AncestorBlock=libraryBase/output
  string : Subsystem  Tag=method provenance  AncestorBlock=libraryBase/output

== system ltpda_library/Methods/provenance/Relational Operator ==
  eq : Subsystem  Tag=method provenance  AncestorBlock=libraryBase/function
  ne : Subsystem  Tag=method provenance  AncestorBlock=libraryBase/function

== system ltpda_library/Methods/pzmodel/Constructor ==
  pzmodel : Subsystem  Tag=method pzmodel  AncestorBlock=libraryBase/constructor

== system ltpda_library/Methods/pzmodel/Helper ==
  get : Subsystem  Tag=method pzmodel  AncestorBlock=libraryBase/function
  isfield : Subsystem  Tag=method pzmodel  AncestorBlock=libraryBase/function
  isvalid : Subsystem  Tag=method pzmodel  AncestorBlock=libraryBase/function
  set : Subsystem  Tag=method pzmodel  AncestorBlock=libraryBase/function
  string : Subsystem  Tag=method pzmodel  AncestorBlock=libraryBase/function

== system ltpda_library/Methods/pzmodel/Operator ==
  tomfir : Subsystem  Tag=method pzmodel  AncestorBlock=libraryBase/function
  tomiir : Subsystem  Tag=method pzmodel  AncestorBlock=libraryBase/function

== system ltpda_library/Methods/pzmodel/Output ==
  char : Subsystem  Tag=method pzmodel  AncestorBlock=libraryBase/output
  display : Subsystem  Tag=method pzmodel  AncestorBlock=libraryBase/output
  save : Subsystem  Tag=method pzmodel  AncestorBlock=libraryBase/output

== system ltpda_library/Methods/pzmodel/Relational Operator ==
  eq : Subsystem  Tag=method pzmodel  AncestorBlock=libraryBase/function
  ne : Subsystem  Tag=method pzmodel  AncestorBlock=libraryBase/function

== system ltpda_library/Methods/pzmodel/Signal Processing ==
  resp : Subsystem  Tag=method pzmodel  AncestorBlock=libraryBase/function

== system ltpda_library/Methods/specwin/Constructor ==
  specwin : Subsystem  Tag=method specwin  AncestorBlock=libraryBase/constructor

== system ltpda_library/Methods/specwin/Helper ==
  get : Subsystem  Tag=method specwin  AncestorBlock=libraryBase/function
  isfield : Subsystem  Tag=method specwin  AncestorBlock=libraryBase/function
  isvalid : Subsystem  Tag=method specwin  AncestorBlock=libraryBase/function
  set : Subsystem  Tag=method specwin  AncestorBlock=libraryBase/function
  string : Subsystem  Tag=method specwin  AncestorBlock=libraryBase/function

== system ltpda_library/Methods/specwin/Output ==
  char : Subsystem  Tag=method specwin  AncestorBlock=libraryBase/output
  display : Subsystem  Tag=method specwin  AncestorBlock=libraryBase/output
  plot : Subsystem  Tag=method specwin  AncestorBlock=libraryBase/output
  save : Subsystem  Tag=method specwin  AncestorBlock=libraryBase/output

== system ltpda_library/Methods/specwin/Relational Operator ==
  eq : Subsystem  Tag=method specwin  AncestorBlock=libraryBase/function
  ne : Subsystem  Tag=method specwin  AncestorBlock=libraryBase/function

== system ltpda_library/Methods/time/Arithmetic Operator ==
  minus : Subsystem  Tag=method time  AncestorBlock=libraryBase/function
  plus : Subsystem  Tag=method time  AncestorBlock=libraryBase/function

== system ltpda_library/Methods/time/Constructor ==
  time : Subsystem  Tag=method time  AncestorBlock=libraryBase/constructor

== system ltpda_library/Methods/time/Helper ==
  get : Subsystem  Tag=method time  AncestorBlock=libraryBase/function
  isfield : Subsystem  Tag=method time  AncestorBlock=libraryBase/function
  isvalid : Subsystem  Tag=method time  AncestorBlock=libraryBase/function
  set : Subsystem  Tag=method time  AncestorBlock=libraryBase/function
  string : Subsystem  Tag=method time  AncestorBlock=libraryBase/function

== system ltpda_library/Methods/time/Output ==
  char : Subsystem  Tag=method time  AncestorBlock=libraryBase/output
  display : Subsystem  Tag=method time  AncestorBlock=libraryBase/output
  format : Subsystem  Tag=method time  AncestorBlock=libraryBase/output
  save : Subsystem  Tag=method time  AncestorBlock=libraryBase/output

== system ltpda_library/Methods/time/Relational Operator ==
  eq : Subsystem  Tag=method time  AncestorBlock=libraryBase/function
  ne : Subsystem  Tag=method time  AncestorBlock=libraryBase/function

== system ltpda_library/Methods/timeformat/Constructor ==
  timeformat : Subsystem  Tag=method timeformat  AncestorBlock=libraryBase/constructor

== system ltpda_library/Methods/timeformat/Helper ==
  get : Subsystem  Tag=method timeformat  AncestorBlock=libraryBase/function
  isfield : Subsystem  Tag=method timeformat  AncestorBlock=libraryBase/function
  isvalid : Subsystem  Tag=method timeformat  AncestorBlock=libraryBase/function
  set : Subsystem  Tag=method timeformat  AncestorBlock=libraryBase/function

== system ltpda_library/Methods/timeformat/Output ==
  char : Subsystem  Tag=method timeformat  AncestorBlock=libraryBase/output
  display : Subsystem  Tag=method timeformat  AncestorBlock=libraryBase/output
  save : Subsystem  Tag=method timeformat  AncestorBlock=libraryBase/output
  string : Subsystem  Tag=method timeformat  AncestorBlock=libraryBase/output

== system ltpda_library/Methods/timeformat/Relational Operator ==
  eq : Subsystem  Tag=method timeformat  AncestorBlock=libraryBase/function
  ne : Subsystem  Tag=method timeformat  AncestorBlock=libraryBase/function

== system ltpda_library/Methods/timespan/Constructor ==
  timespan : Subsystem  Tag=method timespan  AncestorBlock=libraryBase/constructor

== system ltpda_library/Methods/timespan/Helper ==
  get : Subsystem  Tag=method timespan  AncestorBlock=libraryBase/function
  isfield : Subsystem  Tag=method timespan  AncestorBlock=libraryBase/function
  isvalid : Subsystem  Tag=method timespan  AncestorBlock=libraryBase/function
  set : Subsystem  Tag=method timespan  AncestorBlock=libraryBase/function

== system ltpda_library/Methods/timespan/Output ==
  char : Subsystem  Tag=method timespan  AncestorBlock=libraryBase/output
  display : Subsystem  Tag=method timespan  AncestorBlock=libraryBase/output
  save : Subsystem  Tag=method timespan  AncestorBlock=libraryBase/output
  string : Subsystem  Tag=method timespan  AncestorBlock=libraryBase/output

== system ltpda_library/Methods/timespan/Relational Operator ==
  eq : Subsystem  Tag=method timespan  AncestorBlock=libraryBase/function
  ne : Subsystem  Tag=method timespan  AncestorBlock=libraryBase/function

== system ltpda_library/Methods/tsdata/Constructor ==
  tsdata : Subsystem  Tag=method tsdata  AncestorBlock=libraryBase/constructor

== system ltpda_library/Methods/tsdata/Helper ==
  get : Subsystem  Tag=method tsdata  AncestorBlock=libraryBase/function
  isfield : Subsystem  Tag=method tsdata  AncestorBlock=libraryBase/function
  isvalid : Subsystem  Tag=method tsdata  AncestorBlock=libraryBase/function
  set : Subsystem  Tag=method tsdata  AncestorBlock=libraryBase/function

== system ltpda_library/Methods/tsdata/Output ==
  char : Subsystem  Tag=method tsdata  AncestorBlock=libraryBase/output
  display : Subsystem  Tag=method tsdata  AncestorBlock=libraryBase/output
  save : Subsystem  Tag=method tsdata  AncestorBlock=libraryBase/output

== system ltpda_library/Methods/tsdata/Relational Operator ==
  eq : Subsystem  Tag=method tsdata  AncestorBlock=libraryBase/function
  ne : Subsystem  Tag=method tsdata  AncestorBlock=libraryBase/function

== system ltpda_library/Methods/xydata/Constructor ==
  xydata : Subsystem  Tag=method xydata  AncestorBlock=libraryBase/constructor

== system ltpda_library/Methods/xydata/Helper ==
  get : Subsystem  Tag=method xydata  AncestorBlock=libraryBase/function
  isfield : Subsystem  Tag=method xydata  AncestorBlock=libraryBase/function
  isvalid : Subsystem  Tag=method xydata  AncestorBlock=libraryBase/function
  set : Subsystem  Tag=method xydata  AncestorBlock=libraryBase/function

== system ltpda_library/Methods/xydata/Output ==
  char : Subsystem  Tag=method xydata  AncestorBlock=libraryBase/output
  display : Subsystem  Tag=method xydata  AncestorBlock=libraryBase/output
  save : Subsystem  Tag=method xydata  AncestorBlock=libraryBase/output

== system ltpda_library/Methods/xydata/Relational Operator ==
  eq : Subsystem  Tag=method xydata  AncestorBlock=libraryBase/function
  ne : Subsystem  Tag=method xydata  AncestorBlock=libraryBase/function

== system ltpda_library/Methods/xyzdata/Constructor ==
  xyzdata : Subsystem  Tag=method xyzdata  AncestorBlock=libraryBase/constructor

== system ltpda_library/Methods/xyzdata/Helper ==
  get : Subsystem  Tag=method xyzdata  AncestorBlock=libraryBase/function
  isfield : Subsystem  Tag=method xyzdata  AncestorBlock=libraryBase/function
  isvalid : Subsystem  Tag=method xyzdata  AncestorBlock=libraryBase/function
  set : Subsystem  Tag=method xyzdata  AncestorBlock=libraryBase/function

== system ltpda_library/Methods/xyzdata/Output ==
  display : Subsystem  Tag=method xyzdata  AncestorBlock=libraryBase/output
  save : Subsystem  Tag=method xyzdata  AncestorBlock=libraryBase/output

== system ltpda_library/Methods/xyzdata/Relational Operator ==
  eq : Subsystem  Tag=method xyzdata  AncestorBlock=libraryBase/function
  ne : Subsystem  Tag=method xyzdata  AncestorBlock=libraryBase/function

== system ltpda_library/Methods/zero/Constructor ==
  zero : Subsystem  Tag=method zero  AncestorBlock=libraryBase/constructor

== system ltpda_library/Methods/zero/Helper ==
  cat : Subsystem  Tag=method zero  AncestorBlock=libraryBase/function
  get : Subsystem  Tag=method zero  AncestorBlock=libraryBase/function
  isfield : Subsystem  Tag=method zero  AncestorBlock=libraryBase/function
  isvalid : Subsystem  Tag=method zero  AncestorBlock=libraryBase/function
  set : Subsystem  Tag=method zero  AncestorBlock=libraryBase/function
  string : Subsystem  Tag=method zero  AncestorBlock=libraryBase/function

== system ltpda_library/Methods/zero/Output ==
  char : Subsystem  Tag=method zero  AncestorBlock=libraryBase/output
  display : Subsystem  Tag=method zero  AncestorBlock=libraryBase/output
  save : Subsystem  Tag=method zero  AncestorBlock=libraryBase/output

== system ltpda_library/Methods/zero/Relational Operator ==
  eq : Subsystem  Tag=method zero  AncestorBlock=libraryBase/function
  ne : Subsystem  Tag=method zero  AncestorBlock=libraryBase/function

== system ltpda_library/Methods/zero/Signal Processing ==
  resp : Subsystem  Tag=method zero  AncestorBlock=libraryBase/function

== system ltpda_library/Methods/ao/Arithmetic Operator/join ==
  In1 : Inport  OutDataType=sfix(16)  OutScaling=2^0
  join : M-S-Function  Tag=join  FunctionName=ltpdasim
  Out1 : Outport  OutDataType=sfix(16)  OutScaling=2^0
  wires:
  In1/1 -> join/1
  join/1 -> Out1/1

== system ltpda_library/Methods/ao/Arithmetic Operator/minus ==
  In1 : Inport  OutDataType=sfix(16)  OutScaling=2^0
  minus : M-S-Function  Tag=minus  FunctionName=ltpdasim
  Out1 : Outport  OutDataType=sfix(16)  OutScaling=2^0
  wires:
  In1/1 -> minus/1
  minus/1 -> Out1/1

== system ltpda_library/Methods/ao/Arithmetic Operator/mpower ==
  In1 : Inport  OutDataType=sfix(16)  OutScaling=2^0
  mpower : M-S-Function  Tag=mpower  FunctionName=ltpdasim
  Out1 : Outport  OutDataType=sfix(16)  OutScaling=2^0
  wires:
  In1/1 -> mpower/1
  mpower/1 -> Out1/1

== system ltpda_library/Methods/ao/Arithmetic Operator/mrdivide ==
  In1 : Inport  OutDataType=sfix(16)  OutScaling=2^0
  mrdivide : M-S-Function  Tag=mrdivide  FunctionName=ltpdasim
  Out1 : Outport  OutDataType=sfix(16)  OutScaling=2^0
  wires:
  In1/1 -> mrdivide/1
  mrdivide/1 -> Out1/1

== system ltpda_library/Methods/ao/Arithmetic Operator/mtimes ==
  In1 : Inport  OutDataType=sfix(16)  OutScaling=2^0
  mtimes : M-S-Function  Tag=mtimes  FunctionName=ltpdasim
  Out1 : Outport  OutDataType=sfix(16)  OutScaling=2^0
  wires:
  In1/1 -> mtimes/1
  mtimes/1 -> Out1/1

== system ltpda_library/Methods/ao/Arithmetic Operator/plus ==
  In1 : Inport  OutDataType=sfix(16)  OutScaling=2^0
  plus : M-S-Function  Tag=plus  FunctionName=ltpdasim
  Out1 : Outport  OutDataType=sfix(16)  OutScaling=2^0
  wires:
  In1/1 -> plus/1
  plus/1 -> Out1/1

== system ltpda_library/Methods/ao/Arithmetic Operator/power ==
  In1 : Inport  OutDataType=sfix(16)  OutScaling=2^0
  power : M-S-Function  Tag=power  FunctionName=ltpdasim
  Out1 : Outport  OutDataType=sfix(16)  OutScaling=2^0
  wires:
  In1/1 -> power/1
  power/1 -> Out1/1

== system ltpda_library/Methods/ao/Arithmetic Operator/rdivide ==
  In1 : Inport  OutDataType=sfix(16)  OutScaling=2^0
  rdivide : M-S-Function  Tag=rdivide  FunctionName=ltpdasim
  Out1 : Outport  OutDataType=sfix(16)  OutScaling=2^0
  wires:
  In1/1 -> rdivide/1
  rdivide/1 -> Out1/1

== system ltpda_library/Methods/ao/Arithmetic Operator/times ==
  In1 : Inport  OutDataType=sfix(16)  OutScaling=2^0
  times : M-S-Function  Tag=times  FunctionName=ltpdasim
  Out1 : Outport  OutDataType=sfix(16)  OutScaling=2^0
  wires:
  In1/1 -> times/1
  times/1 -> Out1/1

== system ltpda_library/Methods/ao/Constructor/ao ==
  Constant : Constant  OutDataType=sfix(16)  OutScaling=2^0
  ao : M-S-Function  Tag=ao  FunctionName=ltpdasim
  Out1 : Outport  OutDataType=sfix(16)  OutScaling=2^0
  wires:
  Constant/1 -> ao/1
  ao/1 -> Out1/1

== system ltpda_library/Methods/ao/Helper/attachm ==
  In1 : Inport  OutDataType=sfix(16)  OutScaling=2^0
  attachm : M-S-Function  Tag=attachm  FunctionName=ltpdasim
  Out1 : Outport  OutDataType=sfix(16)  OutScaling=2^0
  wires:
  In1/1 -> attachm/1
  attachm/1 -> Out1/1

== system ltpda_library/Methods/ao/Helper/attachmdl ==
  In1 : Inport  OutDataType=sfix(16)  OutScaling=2^0
  attachmdl : M-S-Function  Tag=attachmdl  FunctionName=ltpdasim
  Out1 : Outport  OutDataType=sfix(16)  OutScaling=2^0
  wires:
  In1/1 -> attachmdl/1
  attachmdl/1 -> Out1/1

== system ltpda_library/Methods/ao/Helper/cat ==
  In1 : Inport  OutDataType=sfix(16)  OutScaling=2^0
  cat : M-S-Function  Tag=cat  FunctionName=ltpdasim
  Out1 : Outport  OutDataType=sfix(16)  OutScaling=2^0
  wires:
  In1/1 -> cat/1
  cat/1 -> Out1/1

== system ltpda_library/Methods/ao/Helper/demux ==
  In1 : Inport  OutDataType=sfix(16)  OutScaling=2^0
  demux : M-S-Function  Tag=demux  FunctionName=ltpdasim
  Out1 : Outport  OutDataType=sfix(16)  OutScaling=2^0
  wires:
  In1/1 -> demux/1
  demux/1 -> Out1/1

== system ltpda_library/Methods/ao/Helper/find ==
  In1 : Inport  OutDataType=sfix(16)  OutScaling=2^0
  find : M-S-Function  Tag=find  FunctionName=ltpdasim
  Out1 : Outport  OutDataType=sfix(16)  OutScaling=2^0
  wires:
  In1/1 -> find/1
  find/1 -> Out1/1

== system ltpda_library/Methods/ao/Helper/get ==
  In1 : Inport  OutDataType=sfix(16)  OutScaling=2^0
  get : M-S-Function  Tag=get  FunctionName=ltpdasim
  Out1 : Outport  OutDataType=sfix(16)  OutScaling=2^0
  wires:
  In1/1 -> get/1
  get/1 -> Out1/1

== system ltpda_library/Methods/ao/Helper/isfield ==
  In1 : Inport  OutDataType=sfix(16)  OutScaling=2^0
  isfield : M-S-Function  Tag=isfield  FunctionName=ltpdasim
  Out1 : Outport  OutDataType=sfix(16)  OutScaling=2^0
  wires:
  In1/1 -> isfield/1
  isfield/1 -> Out1/1
